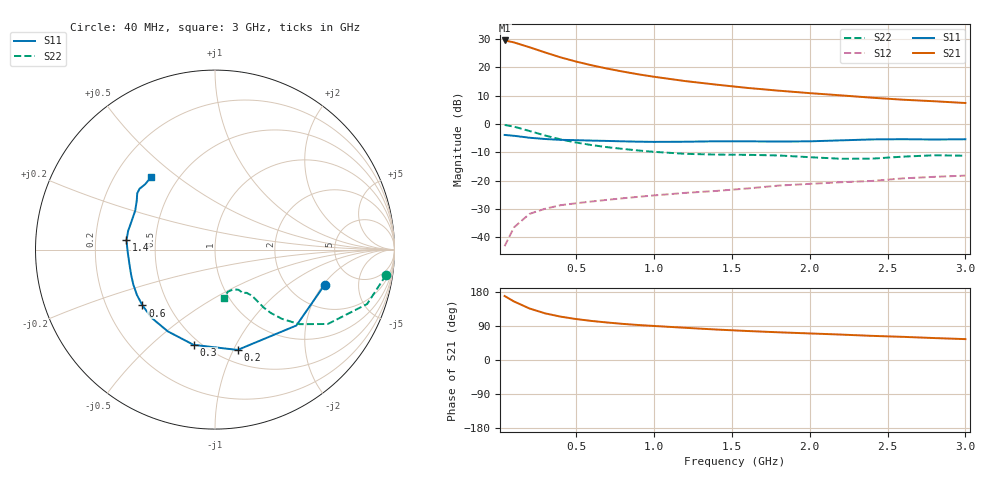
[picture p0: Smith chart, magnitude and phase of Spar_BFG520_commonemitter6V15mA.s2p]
! Filename:  BFG520J.S2P  Version:  2.1
! NXP part #: BFG520  Date: Feb 1992
! Bias condition: Vce=6V, Ic=15mA
! IN LINE PINNING: same data as with cross emitter pinning.
#  MHz  S  MA  R  50
! Freq  S11  S21  S12  S22  !GUM [dB]
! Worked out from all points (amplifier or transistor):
!   21 points, 40 MHz to 3 GHz, reference 50 ohm
!   highest |S21| = 29.5 dB at 40 MHz (marker M1)
!   |S21| within 3 dB of that: start of sweep to 232.7 MHz
!   unconditionally stable (mu >= 1): 1.128 GHz to end of sweep
!   at 300 MHz: K = 0.39, MSG = 27.6 dB, |S12| = -29.9 dB
!   at 1 GHz: K = 0.95, MSG = 20.9 dB, |S12| = -25.2 dB
!   at 3 GHz: K = 1.23, MAG = 9.9 dB, |S12| = -18.2 dB
!   lowest NFmin = 1.30 dB at 500 MHz
!   S11 on the Smith chart (normalised r, x): 40 MHz: 3.11, -2.07; 200 MHz: 0.62, -1.04; 300 MHz: 0.46, -0.69; 600 MHz: 0.36, -0.30; 1.4 GHz: 0.34, +0.05; 3 GHz: 0.35, +0.41
40  0.642 -17.7  29.81 168.9  0.007 80.7  0.964 -8.4
100  0.62 -43.0  27.55 154.5  0.015 71.9  0.9 -19.7
200  0.573 -77.3  22.6 135.9  0.026 60.1  0.753 -33.4
300  0.544 -102.6  18.31 123.1  0.032 53.2  0.627 -41.5
400  0.526 -120.0  14.99 114.4  0.037 51.6  0.536 -46.0
500  0.519 -132.7  12.63 108.0  0.04 50.0  0.471 -48.6
600  0.51 -142.4  10.86 103.0  0.043 50.0  0.425 -49.9
700  0.503 -149.9  9.497 98.9  0.046 50.9  0.39 -50.4
800  0.495 -156.9  8.418 95.3  0.049 52.3  0.364 -50.7
900  0.488 -163.2  7.526 92.3  0.052 54.1  0.341 -51.1
1000  0.484 -168.8  6.819 89.8  0.055 55.5  0.323 -51.7
1200  0.487 -178.8  5.725 85.0  0.061 57.1  0.298 -53.9
1400  0.496 173.9  4.955 80.4  0.066 58.6  0.289 -56.6
1600  0.495 167.9  4.335 76.5  0.073 61.1  0.286 -57.8
1800  0.491 160.9  3.877 73.1  0.082 61.6  0.279 -58.0
2000  0.495 153.8  3.507 70.1  0.088 63.2  0.26 -59.6
2200  0.515 147.8  3.205 67.1  0.094 63.3  0.244 -65.0
2400  0.535 144.1  2.913 63.7  0.099 64.8  0.245 -72.9
2600  0.54 141.1  2.684 61.1  0.11 64.9  0.266 -78.1
2800  0.533 136.9  2.522 57.9  0.117 64.2  0.281 -79.1
3000  0.539 131.1  2.348 55.1  0.123 65.2  0.276 -79.5
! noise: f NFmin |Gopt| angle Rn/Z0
500  1.3  0.256  27  0.25
900  1.45  0.228  52  0.25
1000  1.5  0.233  57  0.28
2000  2.05  0.215  147  0.17
